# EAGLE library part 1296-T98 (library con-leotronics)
1.27mm SINGLE ROW FEMALE SOCKET Source: http://www.leotronics.co.uk/Conexcon/Data%20Sheets/sec.%20A/1296ing.pdf
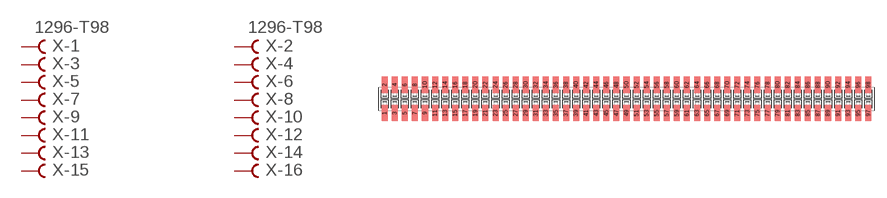
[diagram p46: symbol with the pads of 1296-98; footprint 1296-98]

Designator prefix X; gates -1=FVAL -2=FVAL -3=F -4=F -5=F -6=F -7=F -8=F -9=F -10=F -11=F -12=F -13=F -14=F -15=F -16=F -17=F -18=F -19=F -20=F -21=F -22=F -23=F -24=F -25=F -26=F -27=F -28=F -29=F -30=F -31=F -32=F -33=F -34=F -35=F -36=F -37=F -38=F -39=F -40=F -41=F -42=F -43=F -44=F -45=F -46=F -47=F -48=F -49=F -50=F -51=F -52=F -53=F -54=F -55=F -56=F -57=F -58=F -59=F -60=F -61=F -62=F -63=F -64=F -65=F -66=F -67=F -68=F -69=F -70=F -71=F -72=F -73=F -74=F -75=F -76=F -77=F -78=F -79=F -80=F -81=F -82=F -83=F -84=F -85=F -86=F -87=F -88=F -89=F -90=F -91=F -92=F -93=F -94=F -95=F -96=F -97=F -98=F

## 1296-T98 (OC_FARNELL: unknown; OC_NEWARK: unknown)  [1296-98]
1  -1:B  pas
2  -2:B  pas
3  -3:B  pas
4  -4:B  pas
5  -5:B  pas
6  -6:B  pas
7  -7:B  pas
8  -8:B  pas
9  -9:B  pas
10  -10:B  pas
11  -11:B  pas
12  -12:B  pas
13  -13:B  pas
14  -14:B  pas
15  -15:B  pas
16  -16:B  pas
17  -17:B  pas
18  -18:B  pas
19  -19:B  pas
20  -20:B  pas
21  -21:B  pas
22  -22:B  pas
23  -23:B  pas
24  -24:B  pas
25  -25:B  pas
26  -26:B  pas
27  -27:B  pas
28  -28:B  pas
29  -29:B  pas
30  -30:B  pas
31  -31:B  pas
32  -32:B  pas
33  -33:B  pas
34  -34:B  pas
35  -35:B  pas
36  -36:B  pas
37  -37:B  pas
38  -38:B  pas
39  -39:B  pas
40  -40:B  pas
41  -41:B  pas
42  -42:B  pas
43  -43:B  pas
44  -44:B  pas
45  -45:B  pas
46  -46:B  pas
47  -47:B  pas
48  -48:B  pas
49  -49:B  pas
50  -50:B  pas
51  -51:B  pas
52  -52:B  pas
53  -53:B  pas
54  -54:B  pas
55  -55:B  pas
56  -56:B  pas
57  -57:B  pas
58  -58:B  pas
59  -59:B  pas
60  -60:B  pas
61  -61:B  pas
62  -62:B  pas
63  -63:B  pas
64  -64:B  pas
65  -65:B  pas
66  -66:B  pas
67  -67:B  pas
68  -68:B  pas
69  -69:B  pas
70  -70:B  pas
71  -71:B  pas
72  -72:B  pas
73  -73:B  pas
74  -74:B  pas
75  -75:B  pas
76  -76:B  pas
77  -77:B  pas
78  -78:B  pas
79  -79:B  pas
80  -80:B  pas
81  -81:B  pas
82  -82:B  pas
83  -83:B  pas
84  -84:B  pas
85  -85:B  pas
86  -86:B  pas
87  -87:B  pas
88  -88:B  pas
89  -89:B  pas
90  -90:B  pas
91  -91:B  pas
92  -92:B  pas
93  -93:B  pas
94  -94:B  pas
95  -95:B  pas
96  -96:B  pas
97  -97:B  pas
98  -98:B  pas

## Footprint 1296-98 (pad centres in mm)
1.27mm SINGLE ROW FEMALE SOCKET Source: http://www.leotronics.co.uk/Conexcon/Data%20Sheets/sec.%20A/1296ing.pdf
smd 0.76 x 2.05: 1 -30.48,-1.78; 2 -30.48,1.78; 3 -29.21,-1.78; 4 -29.21,1.78; 5 -27.94,-1.78; 6 -27.94,1.78; 7 -26.67,-1.78; 8 -26.67,1.78; 9 -25.4,-1.78; 10 -25.4,1.78; 11 -24.13,-1.78; 12 -24.13,1.78; 13 -22.86,-1.78; 14 -22.86,1.78; 15 -21.59,-1.78; 16 -21.59,1.78; 17 -20.32,-1.78; 18 -20.32,1.78; 19 -19.05,-1.78; 20 -19.05,1.78; 21 -17.78,-1.78; 22 -17.78,1.78; 23 -16.51,-1.78; 24 -16.51,1.78; 25 -15.24,-1.78; 26 -15.24,1.78; 27 -13.97,-1.78; 28 -13.97,1.78; 29 -12.7,-1.78; 30 -12.7,1.78; 31 -11.43,-1.78; 32 -11.43,1.78; 33 -10.16,-1.78; 34 -10.16,1.78; 35 -8.89,-1.78; 36 -8.89,1.78; 37 -7.62,-1.78; 38 -7.62,1.78; 39 -6.35,-1.78; 40 -6.35,1.78; 41 -5.08,-1.78; 42 -5.08,1.78; 43 -3.81,-1.78; 44 -3.81,1.78; 45 -2.54,-1.78; 46 -2.54,1.78; 47 -1.27,-1.78; 48 -1.27,1.78; 49 0,-1.78; 50 0,1.78; 51 1.27,-1.78; 52 1.27,1.78; 53 2.54,-1.78; 54 2.54,1.78; 55 3.81,-1.78; 56 3.81,1.78; 57 5.08,-1.78; 58 5.08,1.78; 59 6.35,-1.78; 60 6.35,1.78; 61 7.62,-1.78; 62 7.62,1.78; 63 8.89,-1.78; 64 8.89,1.78; 65 10.16,-1.78; 66 10.16,1.78; 67 11.43,-1.78; 68 11.43,1.78; 69 12.7,-1.78; 70 12.7,1.78; 71 13.97,-1.78; 72 13.97,1.78; 73 15.24,-1.78; 74 15.24,1.78; 75 16.51,-1.78; 76 16.51,1.78; 77 17.78,-1.78; 78 17.78,1.78; 79 19.05,-1.78; 80 19.05,1.78; 81 20.32,-1.78; 82 20.32,1.78; 83 21.59,-1.78; 84 21.59,1.78; 85 22.86,-1.78; 86 22.86,1.78; 87 24.13,-1.78; 88 24.13,1.78; 89 25.4,-1.78; 90 25.4,1.78; 91 26.67,-1.78; 92 26.67,1.78; 93 27.94,-1.78; 94 27.94,1.78; 95 29.21,-1.78; 96 29.21,1.78; 97 30.48,-1.78; 98 30.48,1.78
